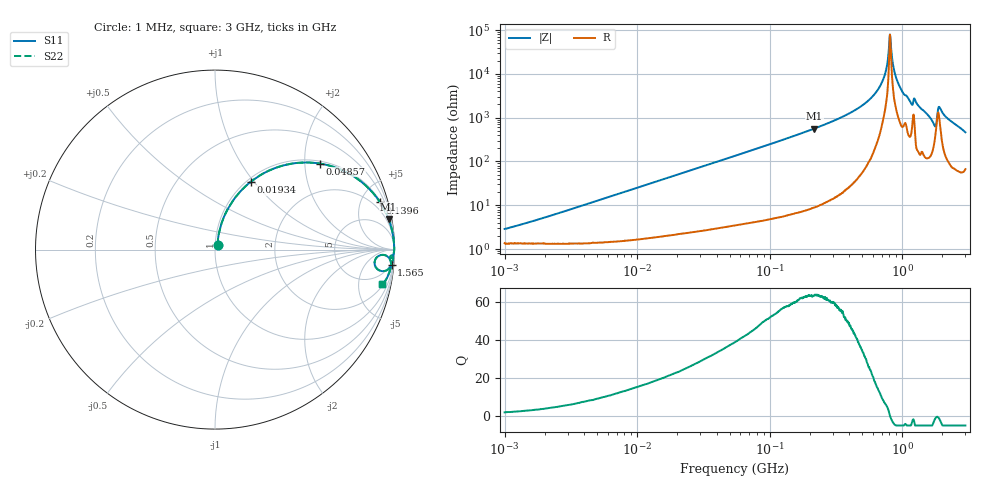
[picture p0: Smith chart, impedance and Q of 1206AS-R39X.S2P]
!s-Parameter Generated by FASTRON Sdn. Bhd.
!FASTRON P/N : 1206AS-R39X
!Keysight Technologies: E4991B_MY54100416_A.01.15
!Date created: Thu Nov 16 11:11:18 2023
!Version  : Rev00 Thu Nov 16 11:11:18 2023
!Data & Calibration Information:
!Freq	S11	S21	S12	S22
!PortZ  Port1:50+j0  Port2:50+j0
!When reading reference impedance value at option line is always used.
! Remarks : This data is being provided solely for informational purposes.
# Hz S dB R 50
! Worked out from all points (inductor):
!   1601 points, 1 MHz to 3 GHz, reference 50 ohm
!   read as one part in series: L = 403 nH near 1.585 MHz
!   highest Q = 63.3 at 216.9 MHz (marker M1), where L = 413 nH
!   self-resonance near 808.6 MHz
!   S11 on the Smith chart (normalised r, x): 1 MHz: 1.03, +0.05; 19.34 MHz: 1.04, +0.96; 48.57 MHz: 1.07, +2.39; 139.6 MHz: 1.12, +6.97; 1.565 GHz: 3, -23; 3 GHz: 2.33, -9.18
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1000000  -30.92 60.3  -0.12 -1.4  -0.12 -1.4  -30.92 60.3
3804036  -20.41 76.7  -0.15 -5.4  -0.15 -5.4  -20.41 76.7
1.447069e7  -9.53 67.5  -0.67 -19.5  -0.67 -19.5  -9.53 67.5
1.934349e7  -7.42 62.3  -1.05 -25.2  -1.05 -25.2  -7.42 62.3
4.857399e7  -2.42 39.3  -3.96 -49.1  -3.96 -49.1  -2.42 39.3
5.477226e7  -2.02 36.1  -4.59 -52.4  -4.59 -52.4  -2.02 36.1
1.396205e8  -0.38 15.9  -11.22 -73.1  -11.22 -73.1  -0.38 15.9
2.083556e8  -0.17 10.5  -14.79 -78.6  -14.79 -78.6  -0.17 10.5
2.168657e8  -0.16 10.0  -15.17 -79.1  -15.17 -79.1  -0.16 10.0
4.0536e8  -0.04 4.4  -22.23 -84.4  -22.23 -84.4  -0.04 4.4
5.870266e8  -0.02 2.0  -29.20 -85.5  -29.20 -85.5  -0.02 2.0
7.207075e8  -0.01 0.7  -37.64 -82.2  -37.64 -82.2  -0.01 0.7
7.539071e8  -0.01 0.5  -41.50 -79.9  -41.50 -79.9  -0.01 0.5
7.925923e8  -0.01 0.2  -50.90 -66.7  -50.90 -66.7  -0.01 0.2
8.249649e8  -0.01 -0.1  -51.85 55.9  -51.85 55.9  -0.01 -0.1
8.892696e8  -0.02 -0.6  -39.31 77.7  -39.31 77.7  -0.02 -0.6
1.002744e9  -0.04 -1.4  -31.89 79.5  -31.89 79.5  -0.04 -1.4
1.159346e9  -0.08 -2.5  -27.03 77.5  -27.03 77.5  -0.08 -2.5
1.565327e9  -0.11 -4.9  -21.31 79.2  -21.31 79.2  -0.11 -4.9
1.747494e9  -0.56 -7.3  -17.15 59.7  -17.15 59.7  -0.56 -7.3
1.931433e9  -0.22 -3.1  -24.60 63.3  -24.60 63.3  -0.22 -3.1
3e9  -0.45 -11.7  -13.78 70.0  -13.78 70.0  -0.45 -11.7
